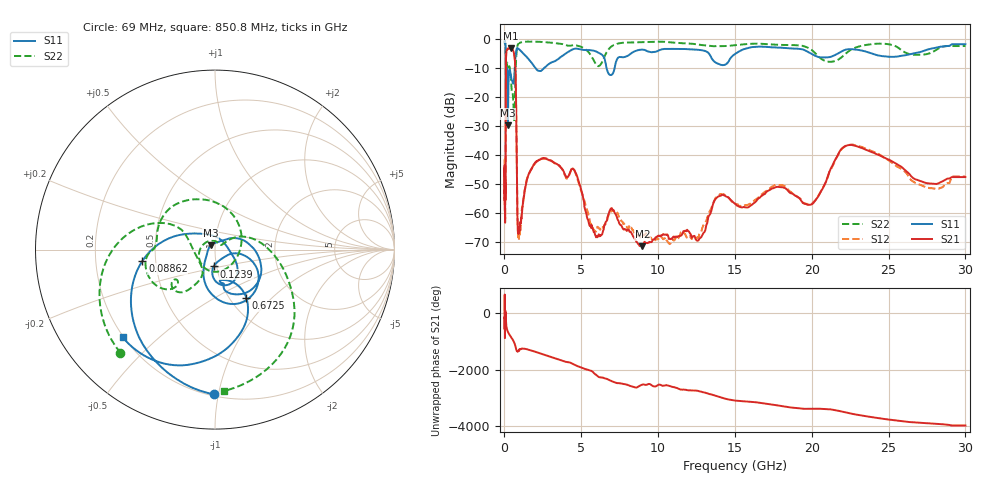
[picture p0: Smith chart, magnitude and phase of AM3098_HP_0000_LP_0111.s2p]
! Date/Time: Thu, Feb 28, 2019 8:30 AM
! Network Analyzer: Agilent Technologies E8364B Rev: A.07.50.67
! Sweep from 0.010 to 30.000 GHz, 1601 Points, Sweep Type: LOG
! Power Supply: 5.023 V, 0.002 A
# Hz S DB R 50
!freq MagS11 AngS11 MagS21 AngS21 MagS12 AngS12 MagS22 AngS22
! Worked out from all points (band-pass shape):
!   1601 points, 10 MHz to 30 GHz, reference 50 ohm
!   highest |S21| = -3.10 dB at 413.9 MHz (marker M1); lowest = -71.3 dB at 8.982 GHz (marker M2)
!   |S21| within 3 dB of the highest: 103.6 MHz to 660.4 MHz (556.9 MHz wide, 146 % of centre)
!   lowest |S11| = -29.6 dB at 225.9 MHz (marker M3), VSWR 1.07, Z = 47.7 + j2.25 ohm
!   |S11| at or under -10 dB: 175.9 MHz to 671.2 MHz (495.3 MHz wide, 117 % of centre); 2.04 GHz to 2.551 GHz (510.8 MHz wide, 22.3 % of centre); 6.649 GHz to 7.164 GHz (515.2 MHz wide, 7.46 % of centre)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
!   |S22| runs from -28.3 to -0.5 dB; largest |S21 - S12| = 0.014
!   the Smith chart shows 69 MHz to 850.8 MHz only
!   S11 on the Smith chart (normalised r, x): 69 MHz: 0.21, -0.97; 88.62 MHz: 0.42, -0.06; 123.9 MHz: 0.97, -0.18; 672.5 MHz: 1.19, -0.71; 850.8 MHz: 0.20, -0.39
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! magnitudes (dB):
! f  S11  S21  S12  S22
! 10 MHz  -0.4  -44.5  -41.4  -0.5
! 38.04 MHz  -0.5  -59.6  -61.3  -0.9
! 69 MHz  -1.9  -52.9  -50.9  -2.1
! 88.62 MHz  -7.8  -19.1  -19.0  -9.1
! 97.94 MHz  -23.9  -7.9  -7.8  -17.4
! 123.9 MHz  -20.5  -4.3  -4.2  -10.7
! 144.7 MHz  -13.0  -3.6  -3.6  -10.1
! 185.8 MHz  -11.4  -3.5  -3.5  -8.1
! 225.9 MHz  -29.6  -3.2  -3.2  -9.4
! 413.9 MHz  -12.4  -3.1  -3.1  -12.9
! 550.5 MHz  -15.1  -3.8  -3.7  -19.3
! 672.5 MHz  -9.9  -6.8  -6.7  -23.5
! 743.2 MHz  -5.0  -16.8  -16.8  -8.4
! 850.8 MHz  -3.0  -62.6  -61.8  -2.0
! 2.084 GHz  -10.3  -42.2  -42.2  -0.8
! 4.503 GHz  -3.3  -44.7  -44.7  -2.0
! 5.959 GHz  -4.1  -68.2  -66.2  -8.6
! 7.926 GHz  -5.9  -65.8  -64.3  -1.1
! 8.982 GHz  -3.5  -71.3  -68.0  -1.0
! 19.8 GHz  -4.4  -57.1  -57.1  -3.0
! 22.67 GHz  -3.4  -36.5  -36.2  -3.2
! 30 GHz  -1.7  -47.5  -47.2  -2.3
